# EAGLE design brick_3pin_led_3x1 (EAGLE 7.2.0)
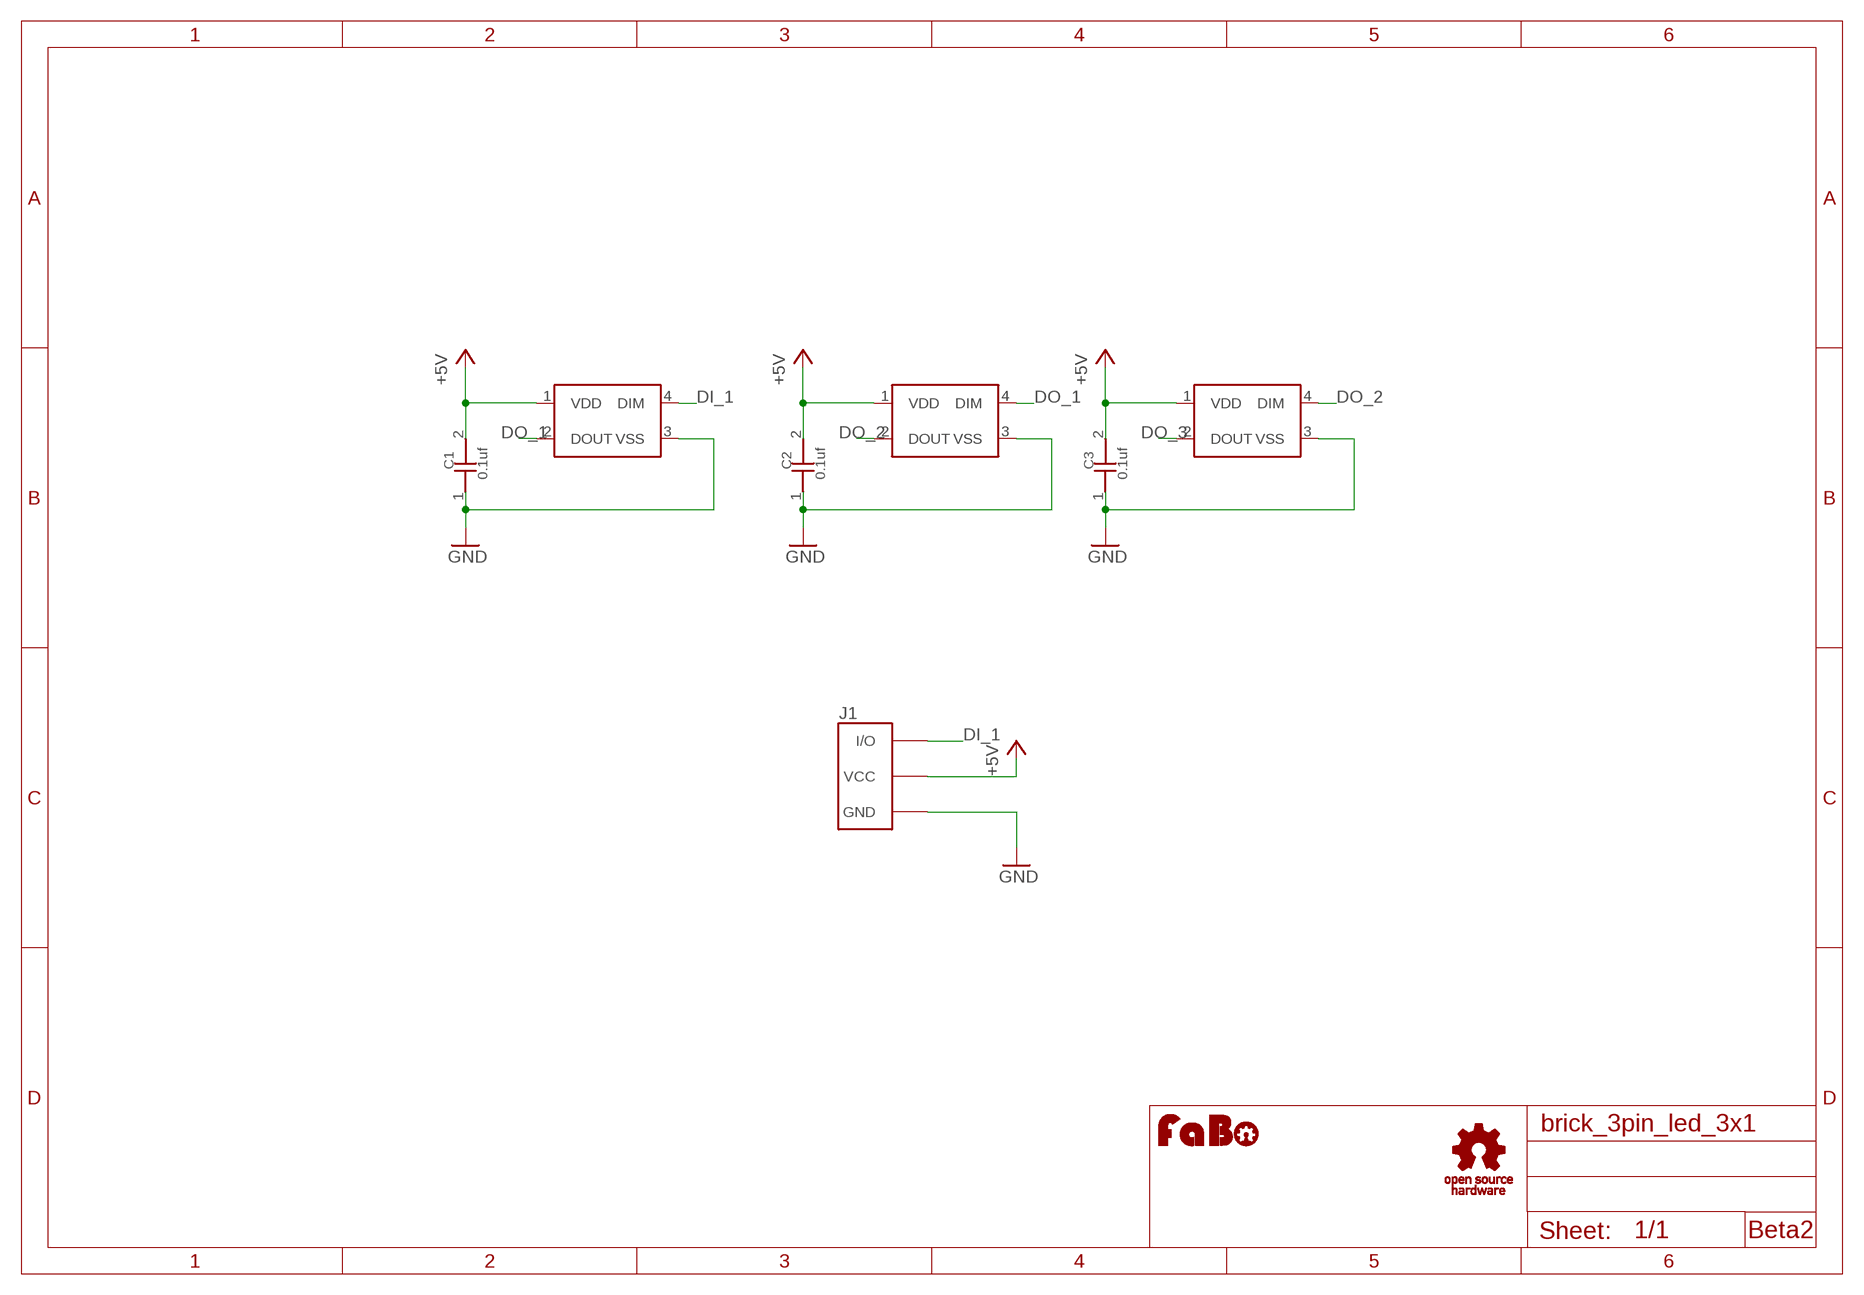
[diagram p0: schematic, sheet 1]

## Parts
C1  0.1uf  CAPACITOR0603  [0603]
C2  0.1uf  CAPACITOR0603  [0603]
C3  0.1uf  CAPACITOR0603  [0603]
J1  BRICK_3PIN_MIDDLE  [BRICK_3PIN_MIDDLE]
LED1  WS2818B  [WS2818B]
LED2  WS2818B  [WS2818B]
LED3  WS2818B  [WS2818B]
U$4  LOGO_FABO-M  [LOGO_FABO_M]
U$5  LOGO_OSHW_T-M  [LOGO_OSHW_T_M]

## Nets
+5V: C1.2 C2.2 C3.2 J1.VCC LED1.1(VDD) LED2.1(VDD) LED3.1(VDD)
DI_1: J1.IN/OUT(I/O) LED1.4(DIM)
DO_1: LED1.2(DOUT) LED2.4(DIM)
DO_2: LED2.2(DOUT) LED3.4(DIM)
DO_3: LED3.2(DOUT)
GND: C1.1 C2.1 C3.1 J1.GND LED1.3(VSS) LED2.3(VSS) LED3.3(VSS)

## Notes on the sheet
- Beta2

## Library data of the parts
C1-C3 = GClue-Capacitor:CAPACITOR
J1 = GClue:BRICK_3PIN: FaBo Brick 3pin
LED1-LED3 = GClue-LED:WS2818B
U$4 = FaBo:LOGO_FABO
U$5 = GClue:LOGO_OSHW_T

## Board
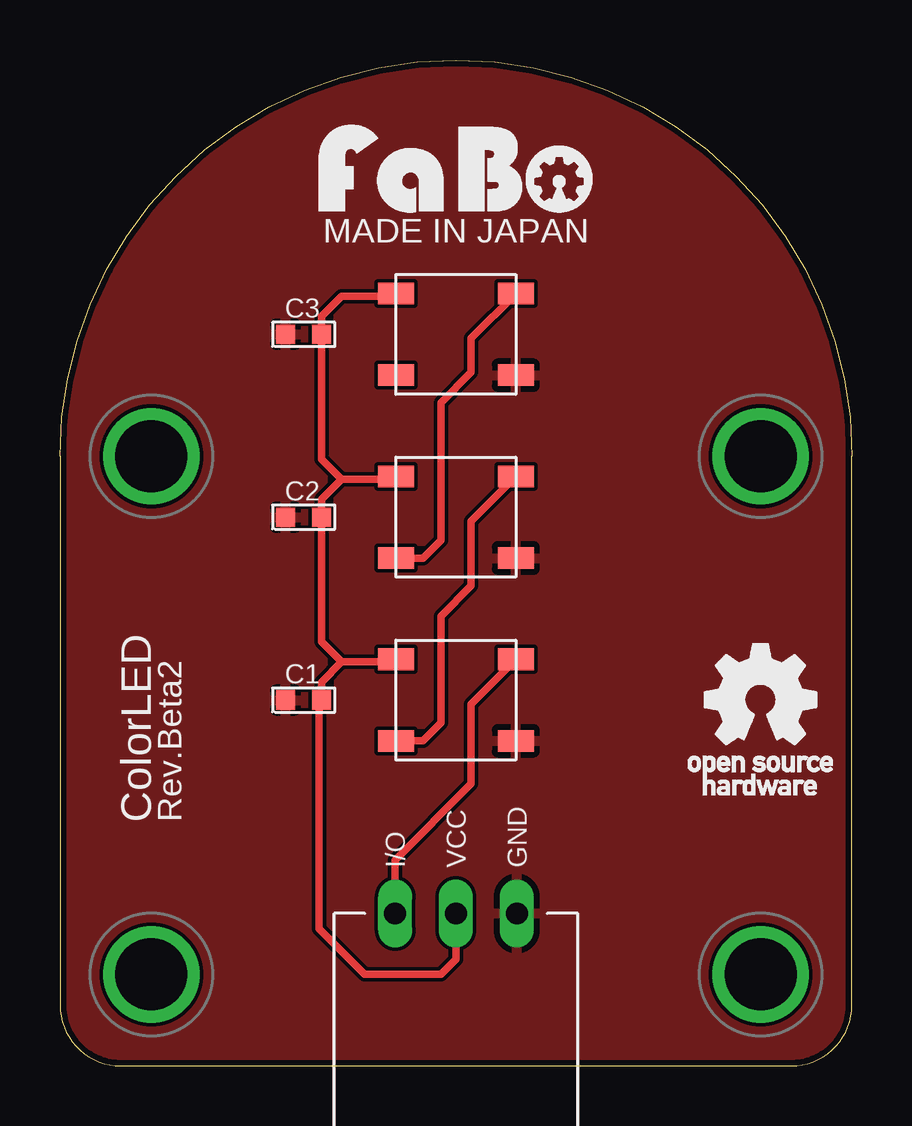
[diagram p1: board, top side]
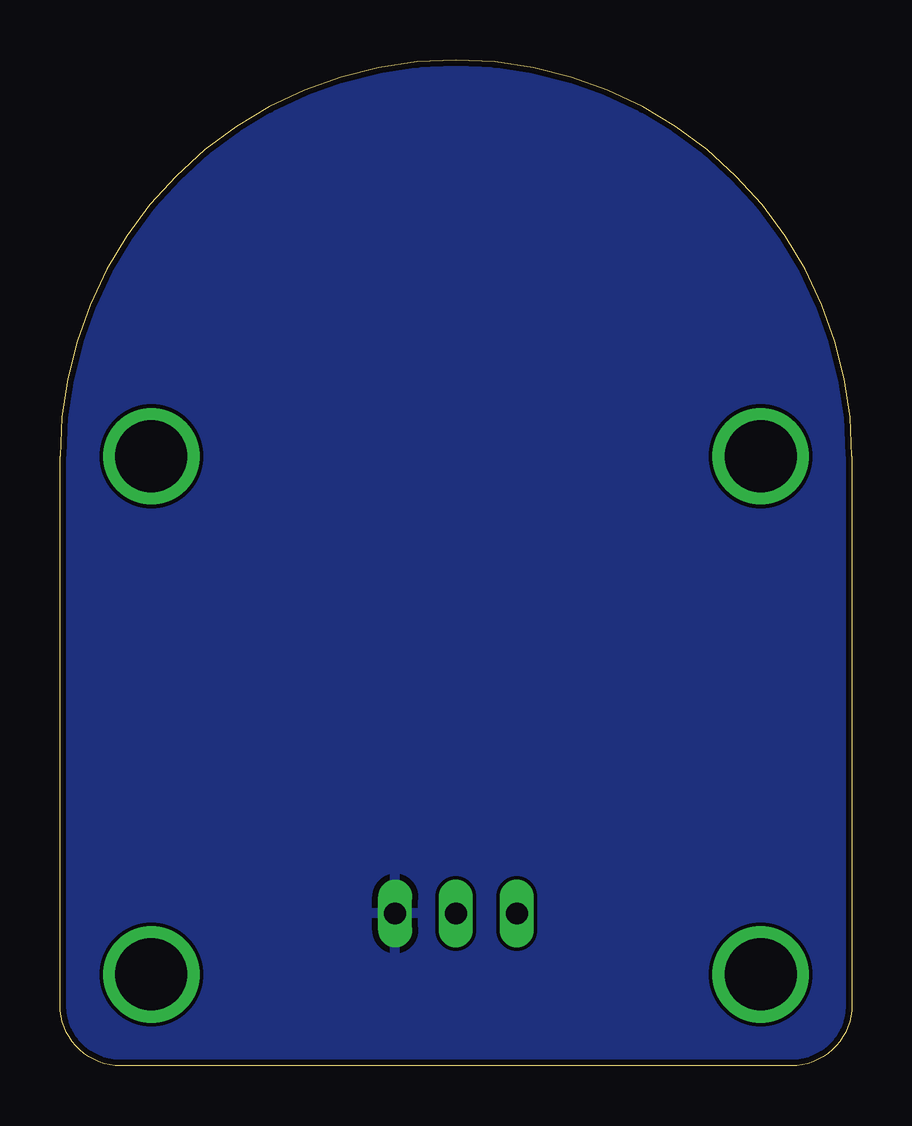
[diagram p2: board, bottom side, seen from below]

Size 33.02 x 41.91 mm. Coordinates in mm from the lower left corner, seen from the top.
Copper layers (1*16): Top 0.035mm / dielectric 1.5mm / Bottom 0.035mm
Design rules "Elecrow_2-layer_eagle_rule": minimum track width 6mil, minimum drill 12mil, track to track 6mil, track to pad 6mil, pad to pad 6mil, via to via 6mil, smd to smd 0mil, copper to edge 10mil, drill to drill 10mil, minimum pad ring 10mil, minimum via ring 6mil, stop-mask expansion 2mil, vias tented up to drill 100mil, thermal gap 10mil

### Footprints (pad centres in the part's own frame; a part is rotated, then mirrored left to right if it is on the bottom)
0603 = smd 0.8 x 0.8: 1 -0.75,0; 2 0.75,0
BRICK_3PIN_MIDDLE = drill 0.9 long: GND 2.54,-8.89; IN/OUT -2.54,-8.89; VCC 0,-8.89 | drill 3 pad 3.81: P$5 -12.7,10.16; P$6 12.7,10.16; P$7 -12.7,-11.43; P$8 12.7,-11.43
WS2818B = smd 1.5 x 0.9: 1 -2.5,1.7; 2 -2.5,-1.7; 3 2.5,-1.7; 4 2.5,1.7

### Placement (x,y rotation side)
C1  10.16,15.24 0 top
C2  10.16,22.86 0 top
C3  10.16,30.48 0 top
J1  16.51,15.24 0 top
LED1  16.51,15.24 0 top
LED2  16.51,22.86 0 top
LED3  16.51,30.48 0 top
U$4  16.51,35.56 0 top
U$5  29.21,15.24 0 top

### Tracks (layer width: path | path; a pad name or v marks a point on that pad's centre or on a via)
+5V
  Top 0.305: J1.VCC 16.51,4.45 15.88,3.81 12.7,3.81 10.79,5.71 10.79,15.12 C1.2 10.91,15.99 11.75,16.83 | 11.75,16.83 13.9,16.83 LED1.1 | 11.75,16.83 10.91,17.66 C2.2 10.91,23.61 11.75,24.45 | 11.75,24.45 13.9,24.45 LED2.1 | 11.75,24.45 10.91,25.29 C3.2 10.91,31.23 11.75,32.07 13.9,32.07 LED3.1
DI_1
  Top 0.305: J1.IN/OUT 13.97,8.57 17.14,11.75 17.14,15.07 LED1.4
DO_1
  Top 0.305: LED1.2 15.13,13.54 15.88,14.29 15.88,18.73 17.14,20 17.14,22.7 LED2.4
DO_2
  Top 0.305: LED2.2 15.13,21.16 15.88,21.91 15.88,27.62 17.14,28.89 17.14,30.32 LED3.4
GND
  pour Bottom: -1.27,-1.27 34.29,-1.27 34.29,43.18 -1.27,43.18
  pour Top: -1.27,-1.27 34.29,-1.27 34.29,43.18 -1.27,43.18

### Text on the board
tPlace: MADE IN JAPAN | ColorLED | Rev.Beta2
